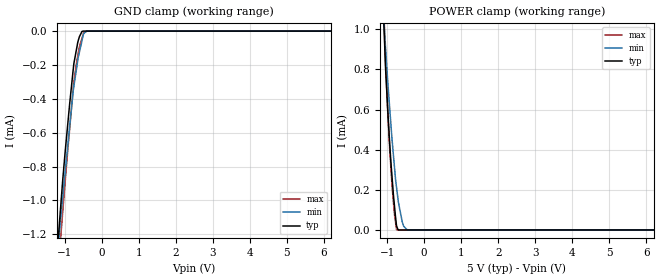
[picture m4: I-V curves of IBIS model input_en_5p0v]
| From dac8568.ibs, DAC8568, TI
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|   INPUT_EN 5.0V Model
[Model]   input_en_5p0v
Model_type   Input
Vinl = 0.4
Vinh = 3.65
|   typ   min   max
|   (nom PVT)   (Fast PVT)  (Slow PVT)
C_comp   4.678e-13   4.324e-13   5.117e-13
|Where nom PVT is Nom process, 3.3V, 25C
|Fast PVT is Strong Process, 3.6V, -40C
|Slow PVT is Weak Process,   3.0V, 125C
[Model Spec]
Vinl   0.4   0.0   0.8
Vinh   3.65   1.8   5.5
[Voltage Range]   5   4.5   5.5
|Juntion temperatures are used in [Temperature Range]
[Temperature Range]   25   125   -40
[Power Clamp Reference]   5   4.5   5.5
[GND Clamp Reference]   0   0   0
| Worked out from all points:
|   GND clamp passes 1 mA (typ) near -1.09 V on its own axis
|   POWER clamp passes 1 mA (typ) near -1.08 V on its own axis
[GND Clamp]
|   Voltage   I(typ)   I(min)   I(max)
-5V       -13.07mA   -10.77mA   -15.7mA
-1.155V   -1.176mA   -1.225mA   -1.362mA
-1.079V   -959.1uA   -1.043mA   -1.144mA
-980mV    -701.4uA   -822.5uA   -876.8uA
-865mV    -433.4uA   -567.4uA   -581.6uA
-750mV    -191.8uA   -326.5uA   -301.4uA
-640mV    -62.78uA   -166.9uA   -140.5uA
-600mV    -32.95uA   -124.6uA   -92.68uA
-530mV    -2.023uA   -56.77uA   -41.2uA
-482mV    0A         -13.73uA   -10.27uA
-401mV    0A         0A         0A
10V       0A         0A         0A
[POWER Clamp]
|   Voltage   I(typ)   I(min)   I(max)
-5V       23.6mA     18.99mA    28.37mA
-1.205V   1.603mA    1.456mA    1.84mA
-1.071V   949.7uA    998.3uA    998.9uA
-1.045V   820uA      918.3uA    851.2uA
-990.5mV  625.8uA    762.3uA    619.7uA
-930mV    429.9uA    606.8uA    402.3uA
-869.5mV  270.3uA    457uA      226.6uA
-809mV    134.8uA    329.6uA    92.56uA
-745mV    20.49uA    210.9uA    1.43uA
-594.5mV  0A         42.58uA    0A
-451.5mV  0A         0A         0A
10V       0A         0A         0A
